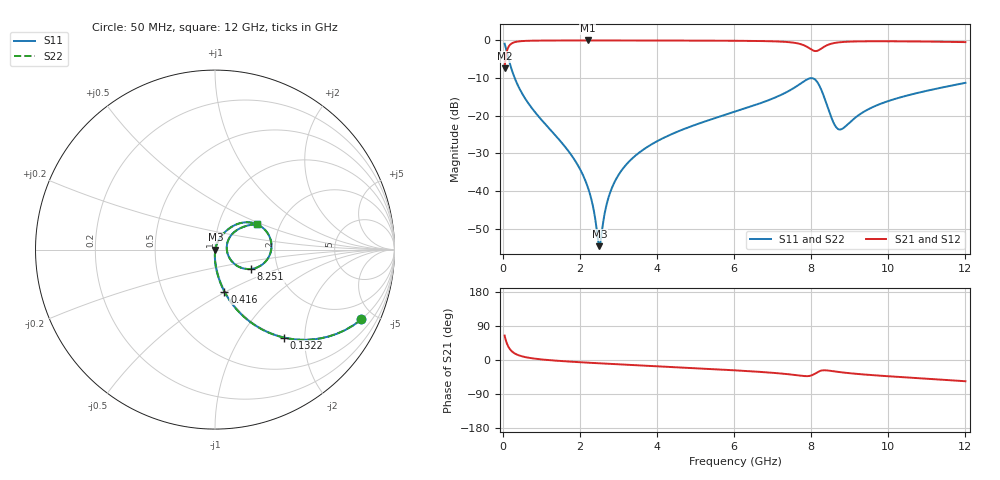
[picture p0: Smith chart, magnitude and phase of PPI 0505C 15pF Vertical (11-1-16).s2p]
# GHz S MA R 50
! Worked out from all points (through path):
!   1601 points, 50 MHz to 12 GHz, reference 50 ohm
!   highest |S21| = -0.02 dB at 2.201 GHz (marker M1); lowest = -7.4 dB at 50 MHz (marker M2)
!   group delay of S21, straight-line fit = 14.6 ps
!   lowest |S11| = -54.6 dB at 2.507 GHz (marker M3), VSWR 1.00, Z = 50.2 - j0.0327 ohm
!   |S11| at or under -10 dB: 312.3 MHz to end of sweep
!   |S22| runs from -54.6 to -0.9 dB; largest |S21 - S12| = 0
!   S11 on the Smith chart (normalised r, x): 50 MHz: 0.99, -4.20; 132.2 MHz: 0.99, -1.59; 416 MHz: 0.99, -0.49; 8.251 GHz: 1.46, -0.33; 12 GHz: 1.52, +0.47
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0.05  0.9039 -25.5  0.4276 64.5  0.4276 64.5  0.9039 -25.5
0.1321563  0.6235 -51.8  0.7814 38.1  0.7814 38.1  0.6235 -51.8
0.2367188  0.4047 -66.9  0.9138 23.0  0.9138 23.0  0.4047 -66.9
0.4159687  0.2401 -77.4  0.9699 12.4  0.9699 12.4  0.2401 -77.4
0.9387813  0.0969 -87.0  0.9941 2.3  0.9941 2.3  0.0969 -87.0
2.044156  0.01795 -90.7  0.998 -6.1  0.998 -6.1  0.01795 -90.7
2.201  0.01156 -88.3  0.998 -7.0  0.998 -7.0  0.01156 -88.3
2.327969  0.006779 -82.4  0.998 -7.7  0.998 -7.7  0.006779 -82.4
2.462406  0.002461 -49.9  0.998 -8.5  0.998 -8.5  0.002461 -49.9
2.507219  0.001864 -10.1  0.998 -8.7  0.998 -8.7  0.001864 -10.1
2.731281  0.007812 65.6  0.9978 -10.0  0.9978 -10.0  0.007812 65.6
2.97775  0.01559 71.2  0.9976 -11.3  0.9976 -11.3  0.01559 71.2
3.403469  0.02844 72.1  0.9972 -13.5  0.9972 -13.5  0.02844 72.1
4.038312  0.04694 70.2  0.9961 -16.7  0.9961 -16.7  0.04694 70.2
6.025  0.1134 60.3  0.9884 -27.3  0.9884 -27.3  0.1134 60.3
7.630781  0.2479 37.6  0.9171 -40.2  0.9171 -40.2  0.2479 37.6
8.019156  0.3156 4.4  0.7501 -40.3  0.7501 -40.3  0.3156 4.4
8.250687  0.2286 -28.1  0.7709 -28.2  0.7709 -28.2  0.2286 -28.1
8.571844  0.08292 -25.3  0.9168 -29.6  0.9168 -29.6  0.08292 -25.3
8.736156  0.06575 2.0  0.9442 -31.9  0.9442 -31.9  0.06575 2.0
10.01331  0.1576 41.9  0.9729 -42.9  0.9729 -42.9  0.1576 41.9
12  0.2734 31.3  0.9484 -56.0  0.9484 -56.0  0.2734 31.3
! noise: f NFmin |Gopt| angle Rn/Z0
0.05  0.0004357  0.8802  1.182  0.0007869
1.372  0.004412  0.701  4.994  0.002885
2.701  0.007325  0.6559  9.384  0.004032
4.031  0.01017  0.6364  13.73  0.005197
5.36  0.01387  0.6461  18.05  0.007251
6.682  0.02343  0.7283  22.57  0.01651
8.012  0.1487  0.9429  27.38  0.5499
9.341  0.0447  0.7975  31.58  0.04236
10.67  0.03509  0.7218  35.37  0.02276
12  0.03907  0.7232  39.28  0.02492
